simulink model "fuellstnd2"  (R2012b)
settings: Solver=ode45  StartTime=0.0  StopTime=10.0  RelTol=1e-3
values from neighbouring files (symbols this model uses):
  A1 = 0.02    [fuellstnd_1.m]    (also in fuellstnd_2.m; fuellstnd_21.m; fuellstnd_3.m; fuellstnd_31.m)
  A12 = 0.005    [fuellstnd_1.m]    (also in fuellstnd_2.m; fuellstnd_21.m; fuellstnd_3.m; fuellstnd_31.m)
  A2 = A1    (= 0.02)    [fuellstnd_1.m]    (also in fuellstnd_2.m; fuellstnd_21.m; fuellstnd_3.m; fuellstnd_31.m)
  A23 = A12    (= 0.005)    [fuellstnd_1.m]    (also in fuellstnd_2.m; fuellstnd_21.m; fuellstnd_3.m; fuellstnd_31.m)
  A3 = A1    (= 0.02)    [fuellstnd_1.m]    (also in fuellstnd_2.m; fuellstnd_21.m; fuellstnd_3.m; fuellstnd_31.m)
  A30 = A12    (= 0.005)    [fuellstnd_1.m]    (also in fuellstnd_2.m; fuellstnd_21.m; fuellstnd_3.m; fuellstnd_31.m)
  D = 0    [aktiv_tilger_1.m]    (also in aktiv_tilger_12.m; aktiv_tilger_3.m = 2000; aktiv_tilger_31.m; beobachter_1.m)
  g = 9.89    [fuellstnd_1.m]    (also in fuellstnd_2.m; fuellstnd_21.m; fuellstnd_3.m; fuellstnd_31.m)
  h10 = 0.0    (= 0)    [fuellstnd_1.m]    (also in fuellstnd_2.m; fuellstnd_21.m; fuellstnd_3.m; fuellstnd_31.m)
  h20 = h10    (= 0)    [fuellstnd_1.m]    (also in fuellstnd_2.m; fuellstnd_21.m; fuellstnd_3.m; fuellstnd_31.m)
  h30 = h10    (= 0)    [fuellstnd_1.m]    (also in fuellstnd_2.m; fuellstnd_21.m; fuellstnd_3.m; fuellstnd_31.m)
  I = 2000    [aktiv_tilger_1.m]    (also in aktiv_tilger_12.m; aktiv_tilger_3.m = 0; aktiv_tilger_31.m = 0; fuellstnd_2.m = 0.0225)
  P = 0    [aktiv_tilger_1.m]    (also in aktiv_tilger_12.m; aktiv_tilger_3.m; aktiv_tilger_31.m; fuellstnd_2.m = 0.09)
  Tp = 1    [fuellstnd_2.m]    (also in fuellstnd_21.m = 0.1; fuellstnd_3.m = 0.1; fuellstnd_31.m = 0.01; regulator_1.m = 5)
  Usoll = 0.4,    [fuellstnd_2.m]    (also in fuellstnd_21.m = 0.2,; fuellstnd_3.m = 0.2,; fuellstnd_31.m = 0.2,)
undefined symbols (not defined in the file or in its folder): sgn
libraries: simulink x1

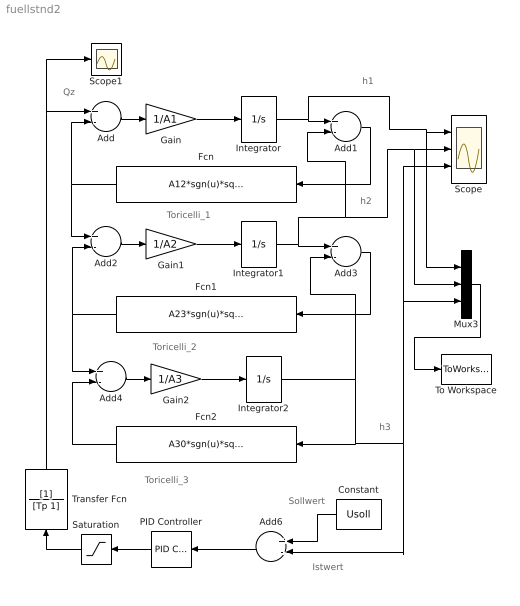
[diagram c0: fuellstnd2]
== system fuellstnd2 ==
  note: Toricelli_3
  note: Istwert
  note: Sollwert
  note: h3
  note: h2
  note: h1
  note: Toricelli_2
  note: Toricelli_1
  note: Qz
  Add{,1..4,6} (6 alike) : Sum  Inputs=+-
  Constant : Constant  Value=Usoll
  Fcn : Fcn  Expr=A12*sgn(u)*sqrt(2*g*abs(u))
  Fcn1 : Fcn  Expr=A23*sgn(u)*sqrt(2*g*abs(u))
  Fcn2 : Fcn  Expr=A30*sgn(u)*sqrt(2*g*abs(u))
  Gain : Gain  Gain=1/A1
  Gain1 : Gain  Gain=1/A2
  Gain2 : Gain  Gain=1/A3
  Integrator : Integrator  InitialCondition=h10
  Integrator1 : Integrator  InitialCondition=h20
  Integrator2 : Integrator  InitialCondition=h30
  Mux3 : Mux  Inputs=3
  PID Controller : simulink/Continuous/PID Controller  Controller=PID  TimeDomain=Continuous-time  SampleTime=1  IntegratorMethod=Forward Euler  FilterMethod=Forward Euler  Form=Parallel  P=P  I=I  D=D  N=100  InitialConditionSource=internal  InitialConditionForIntegrator=0  InitialConditionForFilter=0  ExternalReset=none  LimitOutput=off  UpperSaturationLimit=inf  LowerSaturationLimit=-inf  LinearizeAsGain=on  AntiWindupMode=none  Kb=1  TrackingMode=off  Kt=1  PParamMin=[]  PParamMax=[]  IParamMin=[]  IParamMax=[]  DParamMin=[]  DParamMax=[]  NParamMin=[]  NParamMax=[]  KbParamMin=[]  KbParamMax=[]  KtParamMin=[]  KtParamMax=[]  POutMin=[]  POutMax=[]  IOutMin=[]  IOutMax=[]  DOutMin=[]  DOutMax=[]  NOutMin=[]  NOutMax=[]  KbOutMin=[]  KbOutMax=[]  KtOutMin=[]  KtOutMax=[]  IntegratorOutMin=[]  IntegratorOutMax=[]  FilterOutMin=[]  FilterOutMax=[]  SumOutMin=[]  SumOutMax=[]  SumI1OutMin=[]  SumI1OutMax=[]  SumI2OutMin=[]  SumI2OutMax=[]  SumI3OutMin=[]  SumI3OutMax=[]  SumDOutMin=[]  SumDOutMax=[]  SaturationOutMin=[]  SaturationOutMax=[]  IntegratorContinuousStateAttributes=''  IntegratorStateMustResolveToSignalObject=off  IntegratorRTWStateStorageClass=Auto  FilterContinuousStateAttributes=''  FilterStateMustResolveToSignalObject=off  FilterRTWStateStorageClass=Auto
  Saturation : Saturate  UpperLimit=0.03  LowerLimit=0
  Scope : Scope  NumInputPorts=3
  Scope1 : Scope
  To Workspace : ToWorkspace  VariableName=y  SampleTime=-1  SaveFormat=Structure With Time
  Transfer Fcn : TransferFcn  Denominator=[Tp 1]
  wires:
  Add/1 -> Gain/1
  Gain/1 -> Integrator/1
  Add1/1 -> Fcn/1
  Fcn/1 -> Add/2, Add2/1
  Add2/1 -> Gain1/1
  Gain1/1 -> Integrator1/1
  Fcn1/1 -> Add4/1, Add2/2
  Add4/1 -> Gain2/1
  Gain2/1 -> Integrator2/1
  Fcn2/1 -> Add4/2
  Integrator2/1 -> Fcn2/1, Mux3/3, Scope/3, Add6/2, Add3/2
  Mux3/1 -> To Workspace/1
  Transfer Fcn/1 -> Scope1/1, Add/1
  Integrator1/1 -> Mux3/2, Scope/2, Add1/2, Add3/1
  Integrator/1 -> Mux3/1, Scope/1, Add1/1
  Add6/1 -> PID Controller/1
  Constant/1 -> Add6/1
  PID Controller/1 -> Saturation/1
  Add3/1 -> Fcn1/1
  Saturation/1 -> Transfer Fcn/1
